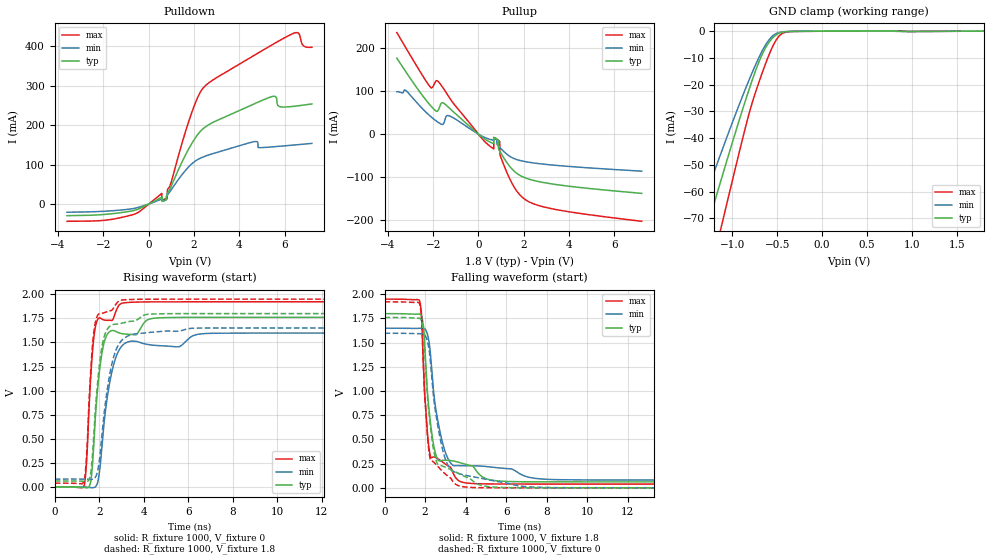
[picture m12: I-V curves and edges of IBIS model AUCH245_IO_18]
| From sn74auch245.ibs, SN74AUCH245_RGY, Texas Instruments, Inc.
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[Model]   AUCH245_IO_18
Model_type  3-state
Enable   Active-Low
Vref =   0
Rref =   1000
Cref =   30p
Vmeas =   0.9
| variable   typ   min   max
C_comp   6.97pF   6.22pF   7.56pF
| C_pullup   7.20pF   1.10pF   11.74pF
| C_pulldown   8.02pF   6.79pF   15.93pF
| C_tri-state   6.97pF   6.22pF   7.56pF
[Temperature Range]   40   100   -40
| Ambient temperature   25   85   -40
[Voltage range]   1.8   1.65   1.95
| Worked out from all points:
|   slope of the pulldown table from 0 to 0.27 V, typ, clamps not added: 34.4 ohm
|   slope of the pullup table from 0 to 0.27 V, typ, clamps not added: 24.5 ohm
|   GND clamp passes 1 mA (typ) near -0.49 V on its own axis
|   rising waveform, R_fixture 1000, V_fixture 0: 20-80 % time 406ps typ, 573ps min, 290ps max; typ from 0 V to 1.76 V
|   falling waveform, R_fixture 1000, V_fixture 1.8: 20-80 % time 464ps typ, 675ps min, 320ps max; typ from 1.8 V to 0.061 V
|   rising waveform, R_fixture 1000, V_fixture 1.8: 20-80 % time 403ps typ, 570ps min, 283ps max; typ from 0.061 V to 1.8 V
|   falling waveform, R_fixture 1000, V_fixture 0: 20-80 % time 473ps typ, 690ps min, 319ps max; typ from 1.76 V to 0 V
[GND Clamp]
| AUCH245_IO_18
|   Voltage   I(typ)   I(min)   I(max)
-3.6V     -348.4mA   -291.7mA   -422.1mA
-1.425V   -90.09mA   -73.63mA   -115.9mA
-1.375V   -84.28mA   -68.86mA   -108.8mA
-1.28V    -73.29mA   -59.88mA   -95.37mA
-1.235V   -68.12mA   -55.66mA   -88.99mA
-1.12V    -55.03mA   -45.02mA   -72.74mA
-825mV    -22.93mA   -19.15mA   -32.24mA
-705mV    -11.58mA   -9.921mA   -19.2mA
-585mV    -3.87mA    -2.962mA   -8.306mA
-460mV    -511uA     -338.7uA   -1.239mA
-330mV    -71.39uA   -55.07uA   -121uA
1.8V      1.088nA    610nA      -1.037nA
[Pulldown]
| AUCH245_IO_18
|   Voltage   I(typ)   I(min)   I(max)
-3.6V     -29.2mA    -20.52mA   -43.49mA
-670mV    -16.37mA   -11.16mA   -26.24mA
580mV     17.79mA    13.06mA    27.14mA
820mV     26.79mA    22.53mA    14.71mA
835mV     27.92mA    23.58mA    37.56mA
1.78V     141.5mA    95.42mA    212mA
2.45V     193.5mA    120.7mA    297.4mA
4.67V     254.7mA    158.8mA    377.9mA
5.45V     273mA      145.2mA    404.3mA
5.76V     247.7mA    146.7mA    414.5mA
6.405V    248.2mA    150mA      433.6mA
7.2V      254.2mA    154.1mA    397.8mA
[Pullup]
| AUCH245_IO_18
|   Voltage   I(typ)   I(min)   I(max)
-3.6V     176.7mA    98.52mA    236.1mA
-2.115V   66.57mA    41.43mA    109mA
-1.775V   55.86mA    27.47mA    122.4mA
-1.53V    71.87mA    25.37mA    105.2mA
-1.29V    60.98mA    42.66mA    85.77mA
510mV     -18.35mA   -12.09mA   -28.08mA
830mV     -11.86mA   -24.61mA   -13.02mA
925mV     -38.3mA    -29.8mA    -16.43mA
955mV     -40.86mA   -31.48mA   -48.18mA
1.26V     -66.43mA   -46.77mA   -89.79mA
2.005V    -100.2mA   -63.13mA   -149.7mA
7.2V      -137.6mA   -85.93mA   -202.4mA
[Ramp]
| AUCH245_IO_18
| variable   typ   min   max
dV/dt_r   1.06/4.07E-10   0.96/5.77E-10   1.16/2.97E-10
dV/dt_f   1.04/4.71E-10   0.94/6.80E-10   1.15/3.24E-10
R_load = 1000
[Rising Waveform]
| AUCH245_IO_18
R_fixture =   1000
C_fixture =   0
L_fixture =   0
V_fixture =   0
V_fixture_min = 0
V_fixture_max = 0
|   Time   V(typ)   V(min)   V(max)
0s        12.09nV    44.84nV    923.4pV
1.33ns    -6.001mV   -550.5uV   19.62mV
1.435ns   -9.662mV   -2.028mV   280.3mV
1.625ns   65.31mV    -7.356mV   1.173V
1.9ns     949.3mV    28.07mV    1.725V
2.295ns   1.554V     820.6mV    1.731V
2.635ns   1.624V     1.261V     1.751V
3.035ns   1.591V     1.468V     1.908V
5.025ns   1.758V     1.463V     1.922V
34.99ns   1.761V     1.597V     1.922V
[Falling Waveform]
| AUCH245_IO_18
R_fixture =   1000
C_fixture =   0
L_fixture =   0
V_fixture =   1.8
V_fixture_min = 1.65
V_fixture_max = 1.95
|   Time   V(typ)   V(min)   V(max)
0s        1.8V       1.65V      1.95V
1.72ns    1.797V     1.649V     1.939V
1.82ns    1.776V     1.65V      1.801V
1.915ns   1.677V     1.65V      1.288V
2.26ns    683.3mV    1.393V     326.4mV
2.5ns     366.9mV    856.5mV    315.7mV
2.915ns   284.6mV    425.3mV    259.1mV
3.835ns   253.5mV    228.6mV    58.08mV
6.145ns   65.53mV    197.8mV    39.68mV
34.99ns   61.33mV    80.74mV    39.23mV
[Rising Waveform]
| AUCH245_IO_18
R_fixture =   1000
C_fixture =   0
L_fixture =   0
V_fixture =   1.8
V_fixture_min = 1.65
V_fixture_max = 1.95
|   Time   V(typ)   V(min)   V(max)
0s        61.28mV    80.7mV     39.22mV
1.33ns    57.7mV     80.63mV    67.13mV
1.435ns   56.64mV    79.9mV     348.7mV
1.625ns   155.3mV    77.88mV    1.239V
1.85ns    881.7mV    111.1mV    1.734V
2.235ns   1.569V     796.6mV    1.81V
2.57ns    1.682V     1.28V      1.836V
2.955ns   1.697V     1.507V     1.938V
6.405ns   1.8V       1.649V     1.95V
34.99ns   1.8V       1.65V      1.95V
[Falling Waveform]
| AUCH245_IO_18
R_fixture =   1000
C_fixture =   0
L_fixture =   0
V_fixture =   0
V_fixture_min = 0
V_fixture_max = 0
|   Time   V(typ)   V(min)   V(max)
0s        1.761V     1.597V     1.922V
1.72ns    1.753V     1.593V     1.911V
1.82ns    1.73V      1.592V     1.775V
1.915ns   1.624V     1.59V      1.278V
2.105ns   985.5mV    1.523V     569.2mV
2.255ns   649.1mV    1.322V     295.3mV
2.54ns    285.7mV    752mV      241.9mV
2.885ns   222.8mV    378.4mV    165.6mV
3.715ns   141.3mV    144.9mV    17.73mV
34.99ns   49.97uV    40.04uV    15.07uV
